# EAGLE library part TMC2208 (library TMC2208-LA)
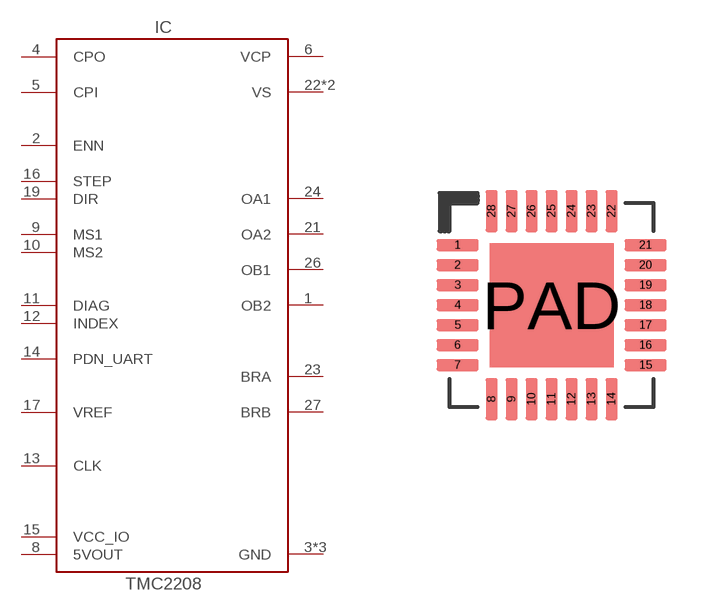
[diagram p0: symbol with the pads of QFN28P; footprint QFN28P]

Designator prefix IC

## TMC2208-LA  [QFN28P]
1  OB2
2  ENN
3  GND
4  CPO
5  CPI
6  VCP
8  5VOUT
9  MS1
10  MS2
11  DIAG
12  INDEX
13  CLK
14  PDN_UART
15  VCC_IO
16  STEP
17  VREF
18  GND
19  DIR
21  OA2
22  VS
23  BRA
24  OA1
26  OB1
27  BRB
28  VS
PAD  GND

## Footprint QFN28P (pad centres in mm)
smd 1.05 x 0.3: 1 -2.35,1.5; 2 -2.35,1; 3 -2.35,0.5; 4 -2.35,0; 5 -2.35,-0.5; 6 -2.35,-1; 7 -2.35,-1.5; 15 2.35,-1.5; 16 2.35,-1; 17 2.35,-0.5; 18 2.35,0; 19 2.35,0.5; 20 2.35,1; 21 2.35,1.5
smd 0.3 x 1.05: 8 -1.5,-2.35; 9 -1,-2.35; 10 -0.5,-2.35; 11 0,-2.35; 12 0.5,-2.35; 13 1,-2.35; 14 1.5,-2.35; 22 1.5,2.35; 23 1,2.35; 24 0.5,2.35; 25 0,2.35; 26 -0.5,2.35; 27 -1,2.35; 28 -1.5,2.35
smd 3.1 x 3.1: PAD 0,0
